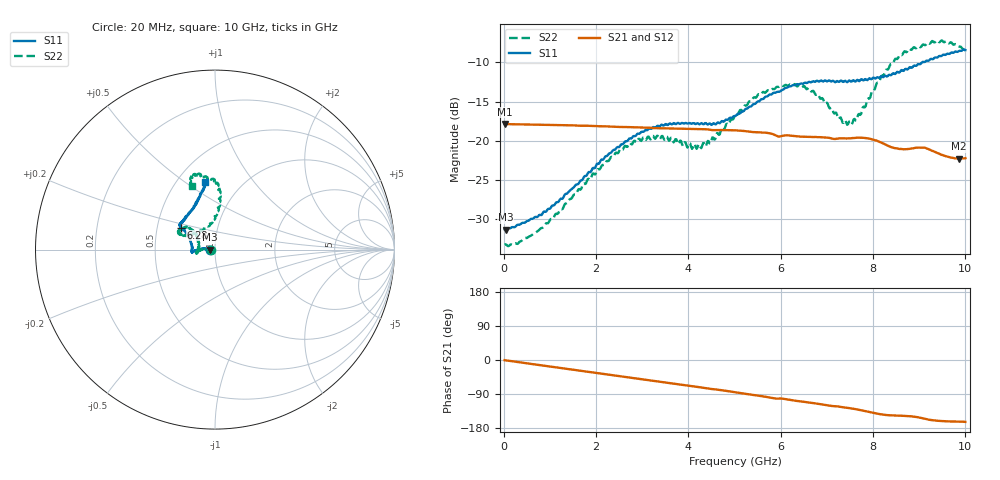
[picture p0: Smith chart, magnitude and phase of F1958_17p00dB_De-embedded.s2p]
! Integrated Device Technology
! Corporate Headquarters
! 6024 Silver Creek Valley Road
! San Jose, CA 95138  USA
! Phone:  1-408-284-8200
! Toll Free:  1-800-223-1366
! Webpage:  http://www.idt.com/
! Timing and RF Division
! 515 Groton Road, Suite 102
! Westford, MA 01886-6024
! Device:  F1958
! Description: 7-bit 0.25 dB Digital Step Attenuator
! Frequency:  0.001 -  6.000 GHz
! Package:  4x4 mm Thin QFN Plastic Package: 24 pin
! Ports:  2 RF, 12 DC
!  Pin  1  = D0
!  Pin  2  = VDD
!  Pin  3  = VMODE
!  Pin  4  = GND
!  Pin  5  = RF1  =  Port 1
!  Pin  6  = GND
!  Pin  7  = GND
!  Pin  8  = GND
!  Pin  9  = GND
!  Pin 10  = GND
!  Pin 11  = GND
!  Pin 12  = GND
!  Pin 13  = GND
!  Pin 14  = RF2  =  Port 2
!  Pin 15  = GND
!  Pin 16  = LE
!  Pin 17  = CLK
!  Pin 18  = DATA
!  Pin 19  = D6
!  Pin 20  = D5
!  Pin 21  = D4
!  Pin 22  = D3
!  Pin 23  = D2
!  Pin 24  = D1
! State:  68
! Atten State:  17.00 dB
! Voltage:  +3.30 Volts
! Current:  0.258 mA
! Data:  The device was measured on a F1958 evaluation board which has
!  individual transmission lines to the RF pins.  Data was collected
!  using a calibrated network analyzer.  The evaluation board was
!  de-embedded using Automatic Fixture Removal (AFR).
!  The reference plane is the edge of the package pin.
! Misc:
!  Action Tracker AT0419
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# GHz S dB R 50
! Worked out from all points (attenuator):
!   500 points, 20 MHz to 10 GHz, reference 50 ohm
!   highest |S21| = -17.87 dB at 20 MHz (marker M1); lowest = -22.3 dB at 9.86 GHz (marker M2)
!   lowest |S11| = -31.4 dB at 40 MHz (marker M3), VSWR 1.06, Z = 47.4 - j0.0676 ohm
!   |S11| at or under -10 dB: start of sweep to 9.058 GHz
!   |S22| runs from -33.5 to -7.2 dB; largest |S21 - S12| = 0.00044
!   S11 on the Smith chart (normalised r, x): 20 MHz: 0.95, -0.00; 6.28 GHz: 0.66, +0.17; 10 GHz: 0.68, +0.60
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0.02  -31.32 -178.4  -17.87 -0.5  -17.87 -0.4  -33.28 -178.2
0.04  -31.36 -178.5  -17.88 -0.8  -17.87 -0.8  -33.23 -177.5
0.32  -30.74 177.0  -17.91 -5.6  -17.91 -5.6  -33.08 177.5
0.84  -29.32 174.9  -17.96 -14.5  -17.95 -14.5  -31.13 178.4
1.7  -25.03 175.8  -18.08 -29.0  -18.08 -29.0  -25.81 177.7
2.6  -20.34 -179.7  -18.25 -44.2  -18.23 -44.3  -20.91 -176.6
2.92  -19.11 -176.6  -18.30 -49.7  -18.29 -49.8  -19.77 -172.9
3.36  -18.16 -173.9  -18.41 -57.1  -18.41 -57.3  -19.65 -168.0
4.26  -17.84 -179.5  -18.52 -72.1  -18.54 -72.2  -20.81 169.9
4.52  -17.91 174.5  -18.65 -76.7  -18.66 -76.8  -19.57 155.1
5.02  -16.84 161.0  -18.67 -85.2  -18.69 -85.2  -16.67 140.4
5.54  -14.95 150.8  -18.93 -94.5  -18.94 -94.4  -14.09 141.7
6.28  -12.89 147.3  -19.39 -106.8  -19.41 -106.8  -12.87 152.5
6.68  -12.46 145.2  -19.53 -113.2  -19.54 -113.2  -13.69 155.5
7.32  -12.34 139.3  -19.71 -124.2  -19.71 -124.1  -17.33 135.7
7.5  -12.36 136.2  -19.70 -127.2  -19.70 -127.1  -17.51 118.0
7.7  -12.40 132.1  -19.60 -131.6  -19.61 -131.5  -16.58 101.0
8.34  -11.59 117.2  -20.68 -145.7  -20.69 -145.9  -10.75 84.0
8.68  -10.96 110.6  -21.09 -147.4  -21.08 -147.4  -8.58 88.2
9.26  -9.54 102.8  -21.24 -158.4  -21.25 -158.5  -7.40 100.7
9.86  -8.55 98.1  -22.29 -162.5  -22.32 -162.5  -7.99 109.5
10  -8.42 98.1  -22.23 -163.3  -22.26 -163.2  -8.47 110.2
